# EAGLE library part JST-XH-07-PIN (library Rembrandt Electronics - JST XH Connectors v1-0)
JST XH Connector 2 Pin Wire to board connector. Pitch: 2,54 mm, (0.100") Number of pins: 7 Created by Rembrandt Electronics www.rembrandtelectronics.com
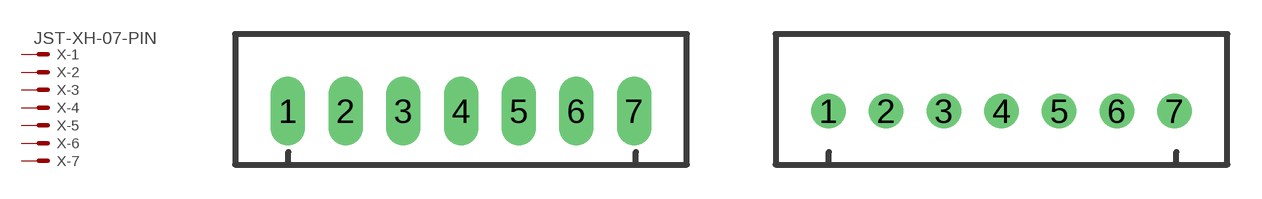
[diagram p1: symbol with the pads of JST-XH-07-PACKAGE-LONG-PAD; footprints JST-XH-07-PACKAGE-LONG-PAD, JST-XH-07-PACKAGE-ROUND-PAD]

Designator prefix X; gates -1=MV -2=M -3=M -4=M -5=M -6=M -7=M

## JST-XH-07-PIN-LONG-PAD  [JST-XH-07-PACKAGE-LONG-PAD]
1  -1:S  pas
2  -2:S  pas
3  -3:S  pas
4  -4:S  pas
5  -5:S  pas
6  -6:S  pas
7  -7:S  pas

## JST-XH-07-PIN-ROUND-PAD  [JST-XH-07-PACKAGE-ROUND-PAD]
Pads as for JST-XH-07-PACKAGE-LONG-PAD

## Footprint JST-XH-07-PACKAGE-LONG-PAD (pad centres in mm)
JST XH Connector Long Pads (Package) Wire to board connector. Pitch: 2,54 mm, (0.100") Number of pins: 7 Created by Rembrandt Electronics www.rembrandtelectronics.com
drill 1.016 long: 1 -7.62,0; 2 -5.08,0; 3 -2.54,0; 4 0,0; 5 2.54,0; 6 5.08,0; 7 7.62,0

## Footprint JST-XH-07-PACKAGE-ROUND-PAD (pad centres in mm)
JST XH Connector Round Pads (Package) Wire to board connector. Pitch: 2,54 mm, (0.100") Number of pins: 7 Created by Rembrandt Electronics www.rembrandtelectronics.com
drill 1.016: 1 -7.62,0; 2 -5.08,0; 3 -2.54,0; 4 0,0; 5 2.54,0; 6 5.08,0; 7 7.62,0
